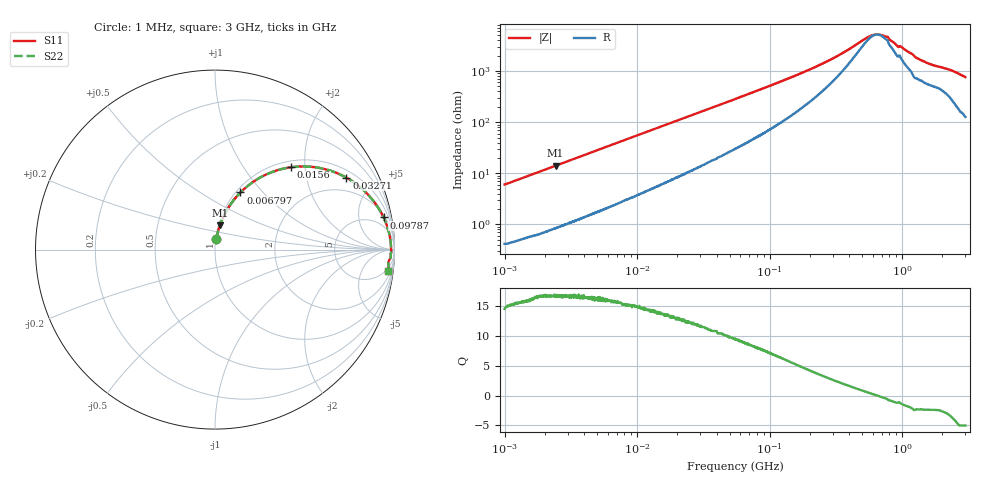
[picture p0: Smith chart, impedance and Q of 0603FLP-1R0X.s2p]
!s-Parameter Generated by FASTRON Sdn. Bhd.
!FASTRON P/N : 0603FLP-1R0X
!Keysight Technologies: E4991B_MY54100416_A.01.15
!Date: Tue Dec 02 12:58:12 2025
!Version  :Rev00  Tue Dec 02 12:58:12 2025
!Data & Calibration Information:
!Freq  S11  S21  S12  S22
!PortZ  Port1:50+j0  Port2:50+j0
!When reading reference impedance value at option line is always used.
! Remarks : This data is being provided solely for informational purposes.
# Hz S dB R 50
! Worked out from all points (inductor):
!   1601 points, 1 MHz to 3 GHz, reference 50 ohm
!   read as one part in series: L = 946 nH near 1.041 MHz
!   highest Q = 16.8 at 2.425 MHz (marker M1), where L = 923 nH
!   self-resonance near 645.5 MHz
!   S11 on the Smith chart (normalised r, x): 1 MHz: 1.01, +0.12; 6.797 MHz: 1.05, +0.76; 15.6 MHz: 1.12, +1.69; 32.71 MHz: 1.31, +3.45; 97.87 MHz: 2, +10; 3 GHz: 4, -15
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1000000  -24.40 82.6  -0.05 -3.4  -0.05 -3.4  -24.40 82.6
2424692  -17.20 78.6  -0.16 -8.0  -0.16 -8.0  -17.20 78.6
3804036  -13.60 74.4  -0.31 -12.1  -0.31 -12.1  -13.60 74.4
6797292  -9.15 66.0  -0.77 -20.4  -0.77 -20.4  -9.15 66.0
9745550  -6.71 58.7  -1.34 -27.4  -1.34 -27.4  -6.71 58.7
1.447069e7  -4.46 49.2  -2.39 -36.7  -2.39 -36.7  -4.46 49.2
1.559866e7  -4.09 47.3  -2.65 -38.5  -2.65 -38.5  -4.09 47.3
2.214172e7  -2.66 38.2  -4.14 -47.2  -4.14 -47.2  -2.66 38.2
3.271304e7  -1.57 28.7  -6.32 -56.2  -6.32 -56.2  -1.57 28.7
5.504702e7  -0.78 18.6  -9.89 -65.4  -9.89 -65.4  -0.78 18.6
9.787053e7  -0.39 10.8  -14.40 -71.2  -14.40 -71.2  -0.39 10.8
2.083556e8  -0.21 4.8  -21.20 -71.2  -21.20 -71.2  -0.21 4.8
3.252521e8  -0.18 2.6  -26.10 -64.0  -26.10 -64.0  -0.18 2.6
5.81181e8  -0.17 0.4  -34.00 -18.6  -34.00 -18.6  -0.17 0.4
6.685918e8  -0.17 -0.1  -34.40 6.5  -34.40 6.5  -0.17 -0.1
7.925923e8  -0.15 -0.8  -32.90 38.0  -32.90 38.0  -0.15 -0.8
9.117997e8  -0.17 -1.4  -30.20 49.1  -30.20 49.1  -0.17 -1.4
9.927591e8  -0.17 -1.6  -29.50 53.3  -29.50 53.3  -0.17 -1.6
1.327057e9  -0.21 -3.0  -25.00 63.8  -25.00 63.8  -0.21 -3.0
1.645649e9  -0.26 -3.8  -22.90 63.5  -22.90 63.5  -0.26 -3.8
2.324278e9  -0.26 -5.1  -20.70 68.8  -20.70 68.8  -0.26 -5.1
3e9  -0.26 -7.2  -17.90 73.2  -17.90 73.2  -0.26 -7.2
